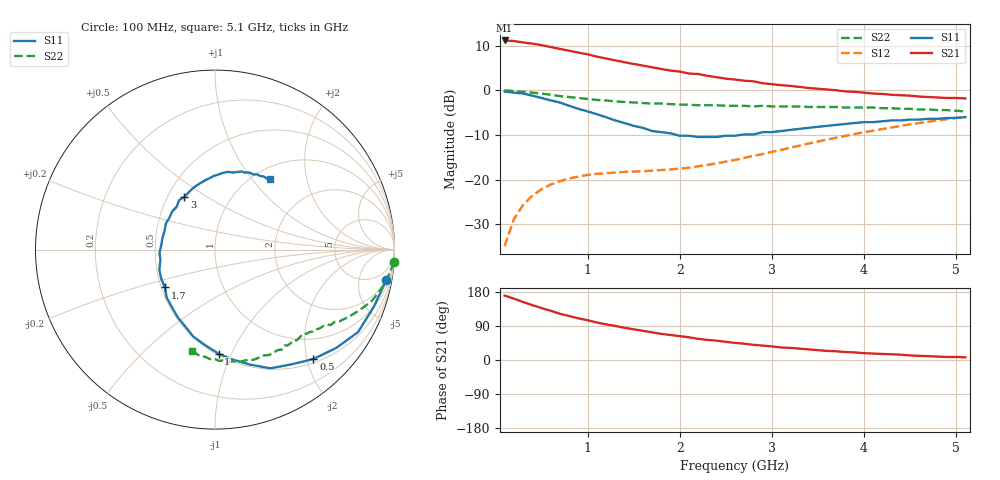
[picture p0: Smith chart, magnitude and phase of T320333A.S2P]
!AT-32033
!S PARAMETERS at Vce=2.7V  Ic=1mA.  LAST UPDATED 01-05-95
# ghz s ma r 50
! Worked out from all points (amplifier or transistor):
!   51 points, 100 MHz to 5.1 GHz, reference 50 ohm
!   highest |S21| = 11.2 dB at 100 MHz (marker M1)
!   |S21| within 3 dB of that: start of sweep to 976.3 MHz
!   unconditionally stable (mu >= 1): 1.907 GHz to 2.823 GHz
!   at 900 MHz: K = 0.51, MSG = 13.9 dB, |S12| = -19.3 dB
!   at 2.6 GHz: K = 1.04, MAG = 7.8 dB, |S12| = -15.6 dB
!   at 5.1 GHz: K = 0.87, MSG = 2.0 dB, |S12| = -5.9 dB
!   S11 on the Smith chart (normalised r, x): 100 MHz: 2, -11; 500 MHz: 0.57, -2.12; 1 GHz: 0.51, -0.89; 1.7 GHz: 0.52, -0.25; 3 GHz: 0.61, +0.40; 5.1 GHz: 1.18, +1.24
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0.1  0.97 -10.0  3.61 170.0  0.018 83.0  1 -4.0
0.2  0.94 -20.0  3.56 162.0  0.036 78.0  0.98 -8.0
0.3  0.92 -30.0  3.43 153.0  0.052 72.0  0.96 -12.0
0.4  0.87 -39.0  3.33 145.0  0.066 67.0  0.94 -15.0
0.5  0.82 -48.0  3.2 137.0  0.078 62.0  0.92 -18.0
0.7  0.73 -65.0  2.9 122.0  0.096 54.0  0.86 -24.0
0.9  0.62 -81.0  2.64 110.0  0.108 49.0  0.82 -28.0
1  0.58 -88.0  2.53 105.0  0.113 47.0  0.8 -30.0
1.1  0.54 -95.0  2.38 99.0  0.116 46.0  0.78 -31.0
1.2  0.5 -104.0  2.27 94.0  0.118 45.0  0.77 -33.0
1.4  0.43 -119.0  2.06 85.0  0.122 44.0  0.74 -35.0
1.7  0.35 -143.0  1.81 73.0  0.126 45.0  0.71 -39.0
1.8  0.34 -152.0  1.73 69.0  0.128 47.0  0.71 -40.0
2.1  0.31 -177.0  1.54 60.0  0.136 51.0  0.69 -44.0
2.2  0.3 175.0  1.52 56.0  0.141 53.0  0.68 -45.0
2.6  0.31 145.0  1.32 45.0  0.166 59.0  0.67 -51.0
2.8  0.32 132.0  1.26 40.0  0.185 61.0  0.66 -54.0
3  0.34 120.0  1.17 36.0  0.205 62.0  0.66 -58.0
3.5  0.39 98.0  1.04 26.0  0.267 62.0  0.65 -67.0
4  0.44 80.0  0.94 18.0  0.339 58.0  0.64 -77.0
4.3  0.46 71.0  0.89 15.0  0.384 54.0  0.63 -84.0
5.1  0.5 52.0  0.81 7.0  0.506 43.0  0.58 -103.0
